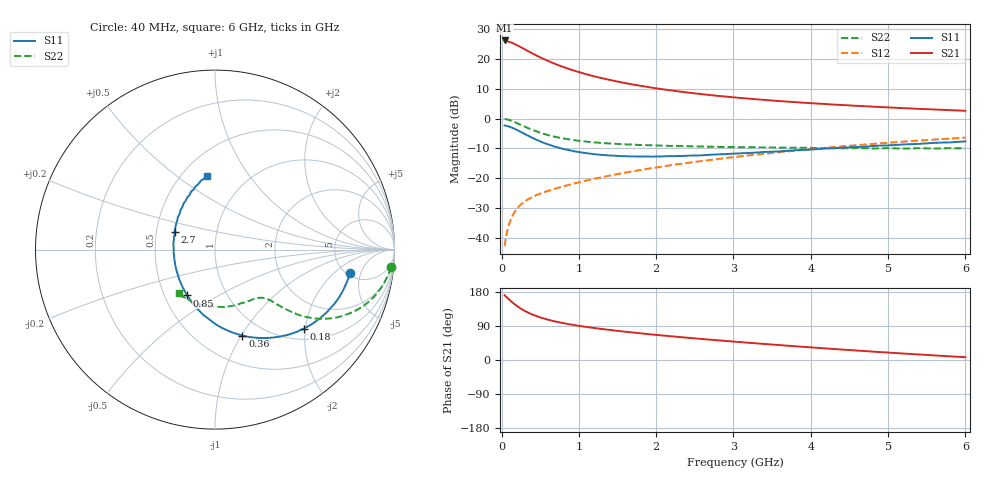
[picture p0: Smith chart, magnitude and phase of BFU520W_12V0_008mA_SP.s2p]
! Filename:  P:\Prog\Test\Noise\ATS_data\Testdata_Net\Run2\BFU520W_APM2013_06_A05_12p0V_008mA_SP_CM01_D.s2p
! Date/Time: Tue 26/Mar/2013 18:01:44
! BFU520W_APM2013_06_A05_12p0V_1to20mA_SP_CM01_Bias5_R.s2p
! MDIF S-parameter v. bias file
! BFU520W_APM2013_06_A05_12p0V_1to20mA_SP_CM01
! Date/time Thu Mar 21 16:35:01 2013
! VAR V_out= 12.0000
! VAR I_out= 7.9950
! VAR V_in= 0.8114
! VAR I_in= 0.0805
! Device data file deembeded for feedlines and parallel
! Original file: \Run2\BFU520W_APM2013_06_A05_12p0V_008mA_SP_CM01_R.s2p
! Feed-files: PR019V01_070313_Feed1.s2p, PR019V01_070313_Feed2.s2p
! Parallel-file: PR019V01_070313_Par.s2p
# MHz S MA R 50
!  Freq-MHz  S11-mag  S11-arg  S21-mag  S21-arg  S12-mag  S12-arg  S22-mag  S22-arg
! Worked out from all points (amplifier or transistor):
!   98 points, 40 MHz to 6 GHz, reference 50 ohm
!   highest |S21| = 26.2 dB at 40 MHz (marker M1)
!   |S21| within 3 dB of that: start of sweep to 303.2 MHz
!   unconditionally stable (mu >= 1): 1.628 GHz to 2.862 GHz
!   at 300 MHz: K = 0.44, MSG = 25.5 dB, |S12| = -27.8 dB
!   at 1.6 GHz: K = 1.00, MSG = 15.0 dB, |S12| = -18.1 dB
!   at 6 GHz: K = 0.88, MSG = 4.5 dB, |S12| = -6.4 dB
!   S11 on the Smith chart (normalised r, x): 40 MHz: 5.31, -3.32; 180 MHz: 1.25, -1.96; 360 MHz: 0.79, -1.01; 850 MHz: 0.65, -0.36; 2.7 GHz: 0.62, +0.13; 6 GHz: 0.66, +0.65
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40  0.7629 -9.9  20.35 171.0  0.007247 83.5  0.9827 -5.6
50  0.7599 -12.3  20.35 168.9  0.008907 82.2  0.98 -7.2
60  0.7546 -14.8  19.97 166.8  0.01064 81.3  0.973 -8.7
80  0.7442 -19.7  19.69 163.0  0.01398 79.4  0.9588 -11.4
120  0.7146 -29.0  18.95 155.6  0.02021 75.4  0.9245 -16.5
180  0.6622 -41.7  17.42 145.7  0.02839 70.3  0.86 -23.0
220  0.6241 -49.6  16.47 139.7  0.03297 67.9  0.8154 -26.4
260  0.5867 -56.6  15.44 134.4  0.03702 65.8  0.7722 -29.4
320  0.5336 -66.5  14.03 127.5  0.0423 63.5  0.7122 -32.8
360  0.5032 -72.3  13.14 123.6  0.04546 62.5  0.6769 -34.5
440  0.4483 -82.8  11.59 116.8  0.05109 61.2  0.6163 -37.0
550  0.3888 -95.0  9.895 109.3  0.05793 60.7  0.551 -39.2
700  0.3354 -109.1  8.167 101.5  0.06704 61.1  0.4917 -40.7
850  0.2987 -121.3  6.926 95.4  0.07601 61.8  0.4515 -41.6
1050  0.268 -135.0  5.749 88.7  0.0882 62.9  0.4165 -42.6
1500  0.2361 -160.4  4.164 76.9  0.1171 64.3  0.3751 -45.8
2050  0.2311 176.5  3.139 65.3  0.1546 64.2  0.3519 -51.4
2700  0.2469 156.0  2.473 53.6  0.202 62.3  0.337 -60.8
3100  0.2616 145.2  2.206 47.1  0.2331 60.5  0.3314 -67.0
4100  0.3086 125.0  1.778 31.9  0.315 54.4  0.3197 -86.0
5200  0.3678 107.3  1.494 17.1  0.4096 45.5  0.3144 -110.1
6000  0.4133 96.3  1.348 7.4  0.4771 38.1  0.3154 -130.0
